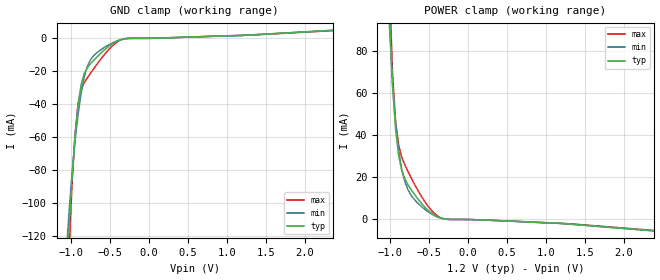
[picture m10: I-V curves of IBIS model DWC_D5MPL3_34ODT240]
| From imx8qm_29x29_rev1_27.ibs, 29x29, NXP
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[Model] DWC_D5MPL3_34ODT240
Model_type   Input
Polarity   Non-Inverting
Enable   Active-High
C_comp   1.266pF   1.183pF   1.367pF
C_comp_power_clamp   289.202fF   266.258fF   313.438fF
C_comp_gnd_clamp 966.831fF   901.511fF   1.047pF
Vinh = 809.000mV
Vinl = 539.000mV
[Model Spec]
D_overshoot_ampl_h 0.35 NA   NA
D_overshoot_ampl_l 0.35 NA   NA
D_overshoot_area_l 100.000p NA   NA
D_overshoot_area_h 100.000p NA   NA
[Receiver Thresholds]
Vth = 674.000mV
Vth_min = 662.000mV
Vth_max = 686.000mV
Vinh_ac = 135.000mV
Vinh_dc = 100.000mV
Vinl_ac = -135.000mV
Vinl_dc = -100.000mV
Tslew_ac = 5.000ns
Reference_supply Power_clamp_ref
[Temperature Range]   25.000   125.000   -40.000
[Voltage Range]   1.200V   1.140V   1.300V
[GND Clamp Reference]   0.00V   0.00V   0.00V
[C Comp Corner]
| variable   typ   min   max
C_comp 1.266pF   1.367pF   1.183pF
C_comp_pullup 289.202fF   313.438fF   266.258fF
C_comp_pulldown 966.831fF   1.047pF   901.511fF
[POWER Clamp Reference]   1.200V   1.140V   1.300V
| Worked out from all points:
|   GND clamp passes 1 mA (typ) near -0.37 V on its own axis
|   POWER clamp passes 1 mA (typ) near -0.38 V on its own axis
[GND Clamp]
-1.182V   -337.6mA   -253.1mA   -424.7mA
-1.064V   -162mA     -136.3mA   -188.8mA
-1.024V   -119.7mA   -107.2mA   -132.8mA
-984.8mV  -86.16mA   -82.97mA   -90.08mA
-945.5mV  -60.11mA   -62.96mA   -59.21mA
-906.1mV  -40.75mA   -46.56mA   -39.91mA
-866.7mV  -28.11mA   -33.45mA   -31.07mA
-787.9mV  -17.91mA   -17.12mA   -24.12mA
-630.3mV  -9.73mA    -7.477mA   -13.61mA
-433.3mV  -2.288mA   -2.086mA   -3.122mA
-315.2mV  -236.5uA   -432.9uA   -218uA
2.364V    4.93mA     4.928mA    4.723mA
[Power Clamp]
-1.164V   361.1mA    266.8mA    463.8mA
-1.006V   97.99mA    91.46mA    110.8mA
-966.7mV  63.78mA    64.72mA    69.28mA
-927.3mV  42.66mA    45.61mA    46.52mA
-887.9mV  30.27mA    32.55mA    35.22mA
-848.5mV  23.31mA    23.79mA    29.6mA
-809.1mV  19.31mA    18mA       26mA
-730.3mV  14.31mA    11.6mA     19.97mA
-533.3mV  5.121mA    4.266mA    7.403mA
-415.1mV  1.611mA    1.634mA    2.362mA
-257.6mV  26.78uA    141.6uA    30.44uA
2.382V    -5.445mA   -5.41mA    -5.222mA
